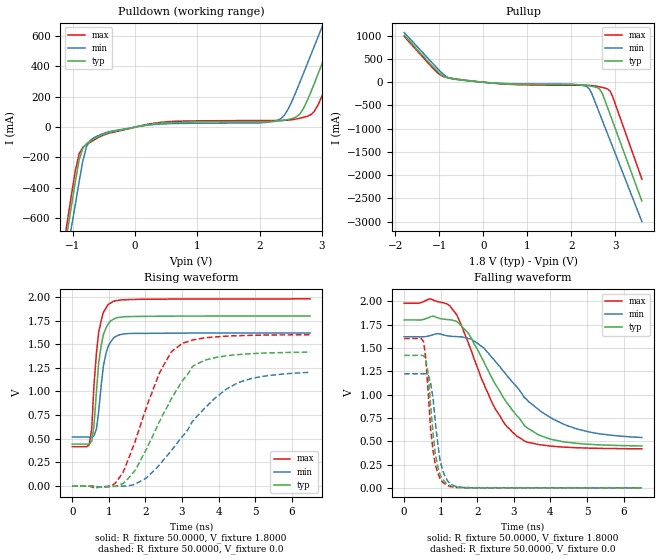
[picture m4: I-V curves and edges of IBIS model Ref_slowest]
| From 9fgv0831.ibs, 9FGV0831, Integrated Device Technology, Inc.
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|   Model Ref_slowest
[Model]  Ref_slowest
Model_type Output
Polarity   Non-Inverting
Enable   Active-High
Vmeas =  0.9000V
Cref =   5.0000pF
Rref =   0.0
Vref =   0.9000V
C_comp   1.1000pF   1.0000pF   1.2000pF
[Temperature Range]   25.0000   75.0000   0.0
[Voltage Range]   1.8000V   1.6200V   1.9800V
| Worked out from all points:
|   slope of the pulldown table from 0 to 0.27 V, typ, clamps not added: 13.6 ohm
|   slope of the pullup table from 0 to 0.27 V, typ, clamps not added: 12.6 ohm
|   rising waveform, R_fixture 50.0000, V_fixture 1.8000: 20-80 % time 204ps typ, 215ps min, 197ps max; typ from 0.444 V to 1.8 V
|   rising waveform, R_fixture 50.0000, V_fixture 0.0: 20-80 % time 1.17ns typ, 1.59ns min, 929ps max; typ from 0 V to 1.42 V
|   falling waveform, R_fixture 50.0000, V_fixture 1.8000: 20-80 % time 1.26ns typ, 1.61ns min, 1.04ns max; typ from 1.8 V to 0.449 V
|   falling waveform, R_fixture 50.0000, V_fixture 0.0: 20-80 % time 216ps typ, 233ps min, 212ps max; typ from 1.42 V to 0 V
[Pulldown]
|Voltage   I(typ)   I(min)   I(max)
-1.8V     -2.523A    -2.538A    -2.518A
-1.14V    -819.8mA   -941.4mA   -756.5mA
-1.02V    -510.3mA   -651.3mA   -436.5mA
-900mV    -218.2mA   -361.2mA   -176.9mA
-780mV    -108.3mA   -127.1mA   -115.2mA
-480mV    -44.15mA   -37.97mA   -48.5mA
2.28V     38.45mA    43.47mA    43.55mA
2.82V     227.8mA    473.1mA    80.46mA
3V        414.1mA    657.2mA    202.9mA
3.24V     664.6mA    902.8mA    452mA
3.42V     852.6mA    1.087A     641.9mA
3.6V      1.04A      1.271A     832mA
[Pullup]
|Voltage   I(typ)   I(min)   I(max)
-1.8V     1.013A     1.068A     986.3mA
-1.08V    265.2mA    331.9mA    235.3mA
-900mV    125.7mA    162.8mA    121.5mA
-780mV    89.6mA     91.86mA    94.5mA
600mV     -39.1mA    -31.81mA   -45.18mA
2.04V     -52.88mA   -43.73mA   -64.93mA
2.28V     -59.25mA   -73.36mA   -65.86mA
2.4V      -74.81mA   -134.8mA   -67.72mA
2.64V     -144.9mA   -673.4mA   -99.02mA
2.7V      -237.1mA   -818.3mA   -112.1mA
2.88V     -697mA     -1.253A    -192.5mA
3.6V      -2.555A    -2.996A    -2.081A
[Ramp]
| variable   typ   min   max
dV/dt_r  0.8496/1.1553n   0.7218/1.6368n   0.9600/0.9274n
dV/dt_f  0.8105/1.2714n   0.6481/1.6528n   0.9368/1.0299n
R_load = 50.0000
[Rising Waveform]
R_fixture= 50.0000
V_fixture= 1.8000
V_fixture_min= 1.6200
V_fixture_max= 1.9800
|time   V(typ)   V(min)   V(max)
0s        443.8mV    518.8mV    416.8mV
460ps     443.3mV    518.1mV    433.7mV
530ps     472.9mV    517.4mV    603.3mV
590ps     629.1mV    530.8mV    1.057V
660ps     1.001V     604.3mV    1.411V
720ps     1.301V     788.8mV    1.625V
850ps     1.603V     1.272V     1.839V
980ps     1.715V     1.48V      1.921V
1.44ns    1.792V     1.611V     1.971V
6.5ns     1.799V     1.619V     1.98V
[Rising Waveform]
R_fixture= 50.0000
V_fixture= 0.0
V_fixture_min= 0.0
V_fixture_max= 0.0
|time   V(typ)   V(min)   V(max)
0s        0V         0V         0V
980ps     -5.443mV   -6.331mV   -4.6mV
1.25ns    5.516mV    -3.117mV   67.56mV
1.71ns    161.4mV    18.76mV    462mV
2.36ns    665.4mV    214.8mV    1.177V
2.69ns    911.4mV    367.9mV    1.412V
3.02ns    1.119V     529mV      1.511V
3.41ns    1.292V     738mV      1.554V
4.46ns    1.388V     1.079V     1.589V
6.5ns     1.416V     1.203V     1.6V
[Falling Waveform]
R_fixture= 50.0000
V_fixture= 1.8000
V_fixture_min= 1.6200
V_fixture_max= 1.9800
|time   V(typ)   V(min)   V(max)
0s        1.8V       1.62V      1.98V
720ps     1.834V     1.634V     2.026V
1.25ns    1.802V     1.626V     1.951V
1.44ns    1.783V     1.621V     1.853V
1.77ns    1.649V     1.6V       1.537V
2.43ns    1.156V     1.386V     891.4mV
2.76ns    939.7mV    1.229V     679.6mV
3.28ns    671.1mV    972.1mV    503.5mV
4.46ns    488.9mV    666.6mV    434.9mV
6.5ns     449.2mV    539.8mV    418.7mV
[Falling Waveform]
R_fixture= 50.0000
V_fixture= 0.0
V_fixture_min= 0.0
V_fixture_max= 0.0
|time   V(typ)   V(min)   V(max)
0s        1.42V      1.223V     1.601V
530ps     1.418V     1.223V     1.57V
590ps     1.375V     1.222V     1.391V
660ps     1.218V     1.204V     1.005V
720ps     899.8mV    1.131V     638.7mV
850ps     367.9mV    712.7mV    251.3mV
980ps     142.1mV    297.5mV    102.1mV
1.18ns    36.79mV    77.39mV    25.59mV
1.58ns    3.249mV    4.626mV    2.2mV
6.5ns     10.76uV    28.53uV    5.246uV
